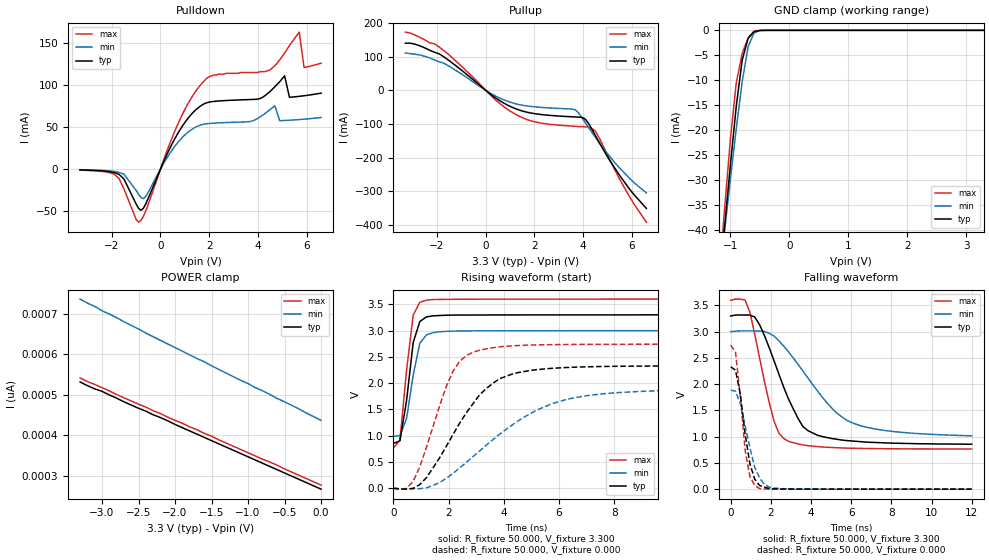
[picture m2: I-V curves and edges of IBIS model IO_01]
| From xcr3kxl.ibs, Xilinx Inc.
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|   Model IO_01
[Model]   IO_01
Model_type   I/O
Polarity   Inverting
Enable   Active-High
Vinl =   0.800V
Vinh =   2.000V
Vmeas =   1.650V
Cref =  50.000pF
Rref =   1.000M
Vref =  0.000V
C_comp   1.250pF   1.000pF   1.500pF
[Temperature Range]   50.000   100.000   0.000
[Voltage Range]   3.300V   3.000V   3.600V
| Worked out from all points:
|   slope of the pulldown table from 0 to 0.495 V, typ, clamps not added: 16 ohm
|   slope of the pullup table from 0 to 0.495 V, typ, clamps not added: 18.3 ohm
|   GND clamp passes 1 mA (typ) near -0.65 V on its own axis
|   rising waveform, R_fixture 50.000, V_fixture 3.300: 20-80 % time 364ps typ, 397ps min, 345ps max; typ from 0.852 V to 3.3 V
|   rising waveform, R_fixture 50.000, V_fixture 0.000: 20-80 % time 1.76ns typ, 2.88ns min, 1.08ns max; typ from 0.001 V to 2.33 V
|   falling waveform, R_fixture 50.000, V_fixture 3.300: 20-80 % time 1.56ns typ, 2.5ns min, 982ps max; typ from 3.3 V to 0.856 V
|   falling waveform, R_fixture 50.000, V_fixture 0.000: 20-80 % time 518ps typ, 700ps min, 451ps max; typ from 2.33 V to 0 V
[Pulldown]
| voltage   I(typ)   I(min)   I(max)
-3.3V     -800uA     -600uA     -1.1mA
-1.7V     -6.1mA     -3.7mA     -11mA
-900mV    -46.35mA   -29.77mA   -62.96mA
-600mV    -41.06mA   -32.32mA   -49.47mA
800mV     46.65mA    34.66mA    59.01mA
1.9V      79mA       54.02mA    108mA
4.5V      92.31mA    70.92mA    118mA
5.1V      111mA      57.94mA    138mA
5.3V      85.46mA    58.26mA    147mA
5.7V      86.62mA    59.04mA    163mA
5.9V      87.32mA    59.5mA     121mA
6.6V      90.4mA     61.49mA    126mA
[Pullup]
| voltage   I(typ)   I(min)   I(max)
-3.3V     140mA      111mA      173mA
-2.9V     137mA      107mA      164mA
-1.9V     108mA      84.43mA    128mA
400mV     -22.34mA   -16.86mA   -28.34mA
1.3V      -56.68mA   -41.29mA   -74.24mA
2.1V      -70.35mA   -49.69mA   -95.08mA
3.6V      -78.94mA   -56.27mA   -107mA
3.8V      -79.64mA   -66.55mA   -108mA
4.1V      -86.5mA    -97.21mA   -109mA
4.5V      -134mA     -139mA     -121mA
5.5V      -253mA     -231mA     -264mA
6.6V      -351mA     -305mA     -392mA
[GND_clamp]
| voltage   I(typ)   I(min)   I(max)
-3.3V     -265mA     -226mA     -304mA
-1.2V     -52.28mA   -50.76mA   -50.82mA
-1.1V     -39.47mA   -40.24mA   -35.9mA
-1V       -26.88mA   -29.77mA   -21.76mA
-900mV    -15.13mA   -19.6mA    -10.45mA
-800mV    -5.967mA   -10.29mA   -4.628mA
-700mV    -1.62mA    -3.333mA   -1.533mA
-600mV    -271uA     -529uA     -194uA
-500mV    -24.86uA   -57.89uA   -10.46uA
-400mV    -1.648uA   -5.395uA   -366nA
3.3V      234pA      465pA      222pA
[POWER_clamp]
| voltage   I(typ)   I(min)   I(max)
-3.3V     532pA      737pA      542pA
-3.2V     523pA      727pA      533pA
-3.1V     515pA      719pA      526pA
-3V       509pA      708pA      518pA
-2.9V     500pA      700pA      510pA
-2.7V     483pA      681pA      493pA
-2.4V     460pA      653pA      470pA
-2.3V     451pA      644pA      461pA
-2.1V     436pA      626pA      445pA
-700mV    323pA      501pA      334pA
-300mV    291pA      465pA      301pA
0V        267pA      437pA      277pA
[Ramp]
| variable   typ   min   max
dV/dt_r   1.397/1.749n   1.126/2.874n   1.644/1.072n
dV/dt_f   1.467/1.560n   1.190/2.493n   1.701/0.977n
R_load = 50.000
[Rising Waveform]
R_fixture = 50.000
V_fixture = 3.300
V_fixture_min = 3.000
V_fixture_max = 3.600
L_fixture = 0.000H
C_fixture = 0.000F
| time   V(typ)   V(min)   V(max)
0s        852mV      987mV      764mV
240ps     903mV      1.002V     915mV
480ps     1.671V     1.327V     2.246V
720ps     2.775V     2.157V     3.294V
960ps     3.173V     2.759V     3.538V
1.2ns     3.261V     2.919V     3.58V
1.44ns    3.281V     2.961V     3.591V
1.92ns    3.293V     2.985V     3.594V
3.12ns    3.297V     2.996V     3.598V
12ns      3.3V       2.999V     3.6V
[Rising Waveform]
R_fixture = 50.000
V_fixture = 0.000
V_fixture_min = 0.000
V_fixture_max = 0.000
L_fixture = 0.000H
C_fixture = 0.000F
| time   V(typ)   V(min)   V(max)
0s        1.111mV    715uV      747uV
480ps     -16.9mV    -13.15mV   -2.796mV
720ps     -412uV     -11.21mV   135mV
1.2ns     203mV      8.659mV    781mV
2.16ns    1.021V     283mV      2.224V
2.88ns    1.604V     599mV      2.586V
3.84ns    2.083V     1.025V     2.691V
5.04ns    2.247V     1.444V     2.726V
6.24ns    2.297V     1.685V     2.736V
12ns      2.329V     1.876V     2.74V
[Falling Waveform]
R_fixture = 50.000
V_fixture = 3.300
V_fixture_min = 3.000
V_fixture_max = 3.600
L_fixture = 0.000H
C_fixture = 0.000F
| time   V(typ)   V(min)   V(max)
0s        3.297V     2.998V     3.597V
720ps     3.315V     3.013V     3.6V
960ps     3.314V     3.013V     3.363V
1.44ns    3.13V      3.011V     2.497V
2.16ns    2.445V     2.914V     1.292V
2.64ns    1.942V     2.724V     965mV
3.84ns    1.116V     2.12V      829mV
5.28ns    950mV      1.447V     789mV
6ns       918mV      1.271V     780mV
12ns      856mV      1.017V     764mV
[Falling Waveform]
R_fixture = 50.000
V_fixture = 0.000
V_fixture_min = 0.000
V_fixture_max = 0.000
L_fixture = 0.000H
C_fixture = 0.000F
| time   V(typ)   V(min)   V(max)
0s        2.329V     1.885V     2.741V
240ps     2.266V     1.867V     2.613V
480ps     1.811V     1.625V     1.774V
720ps     1.053V     1.201V     740mV
960ps     478mV      787mV      237mV
1.2ns     189mV      416mV      71.9mV
1.44ns    70.65mV    213mV      9.725mV
1.92ns    12.37mV    35.89mV    3.172mV
2.4ns     3.477mV    12.74mV    1.707mV
12ns      45.23uV    133uV      26.22uV
